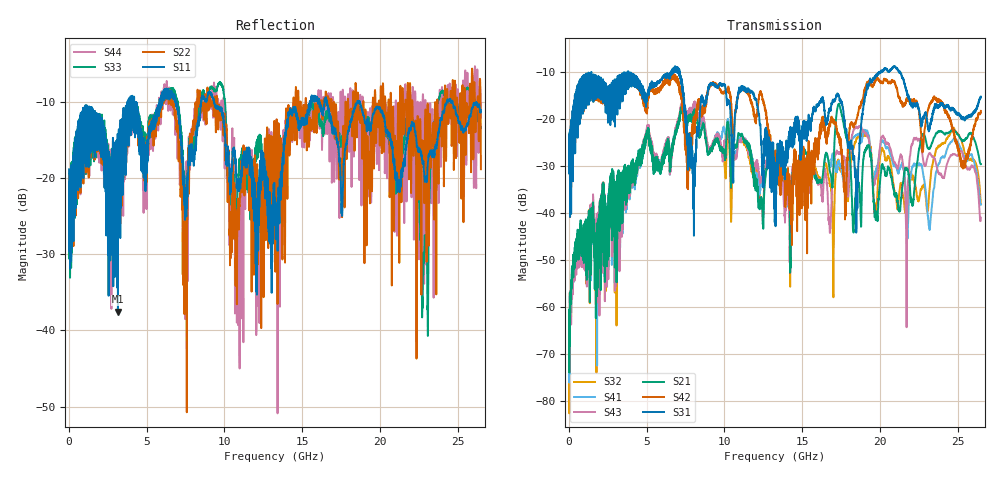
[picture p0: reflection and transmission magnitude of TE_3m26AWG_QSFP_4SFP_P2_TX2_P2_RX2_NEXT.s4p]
!Agilent Technologies,N5222A,MY51421691,A.10.00.00
!Agilent N5222A: A.10.00.00
!Date: Friday, January 30, 2015 12:35:31
!Correction: S11(Full 4 Port(1,2,3,4))
!S12(Full 4 Port(1,2,3,4))
!S13(Full 4 Port(1,2,3,4))
!S14(Full 4 Port(1,2,3,4))
!S21(Full 4 Port(1,2,3,4))
!S22(Full 4 Port(1,2,3,4))
!S23(Full 4 Port(1,2,3,4))
!S24(Full 4 Port(1,2,3,4))
!S31(Full 4 Port(1,2,3,4))
!S32(Full 4 Port(1,2,3,4))
!S33(Full 4 Port(1,2,3,4))
!S34(Full 4 Port(1,2,3,4))
!S41(Full 4 Port(1,2,3,4))
!S42(Full 4 Port(1,2,3,4))
!S43(Full 4 Port(1,2,3,4))
!S44(Full 4 Port(1,2,3,4))
!S4P File: Measurements: <S11,S12,S13,S14>,
!<S21,S22,S23,S24>,
!<S31,S32,S33,S34>,
!<S41,S42,S43,S44>:
# Hz S  dB  R 50.0
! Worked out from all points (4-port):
!   2650 points, 10 MHz to 26.5 GHz, reference 50 ohm
!   strongest paths, dB at 10 MHz, 6.63 GHz, 13.26 GHz, 19.88 GHz, 26.5 GHz:
!     S31: -24.8, -10.2, -30.2, -10.6, -15.3
!     S42: -24.8, -11.4, -30.6, -11.7, -18.3
!     S21: -65.3, -25.9, -29.2, -39.1, -29.7
!     S43: -68.7, -26.3, -29.9, -30.2, -41.0
!     S41: -74.3, -26.0, -30.3, -29.5, -38.2
!     S32: -63.4, -26.0, -31.1, -33.4, -38.2
!   lowest |S11| = -37.5 dB at 3.15 GHz (marker M1), VSWR 1.03, Z = 50.6 - j1.19 ohm
!   |S11| at or under -10 dB: start of sweep to 3.77 GHz; 9.336 GHz to 15.49 GHz (6.159 GHz wide, 49.6 % of centre); 18.72 GHz to 24.3 GHz (5.577 GHz wide, 25.9 % of centre)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
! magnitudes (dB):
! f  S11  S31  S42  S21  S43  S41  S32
! 10 MHz  -18.8  -24.8  -24.8  -65.3  -68.7  -74.3  -63.4
! 3.15 GHz  -37.5  -16.9  -15.7  -31.3  -33.5  -32.2  -32.7
! 7.32 GHz  -20.2  -13.6  -17.2  -16.9  -16.1  -16.6  -16.5
! 18.5 GHz  -10.2  -39.9  -20.1  -34.6  -21.7  -23.5  -24.1
! 20 GHz  -10.8  -10.3  -12.1  -33.9  -26.3  -26.8  -28.6
! 22.76 GHz  -17.9  -20.0  -26.4  -23.2  -28.1  -31.2  -34.5
! 26.5 GHz  -11.0  -15.3  -18.3  -29.7  -41.0  -38.2  -38.2
